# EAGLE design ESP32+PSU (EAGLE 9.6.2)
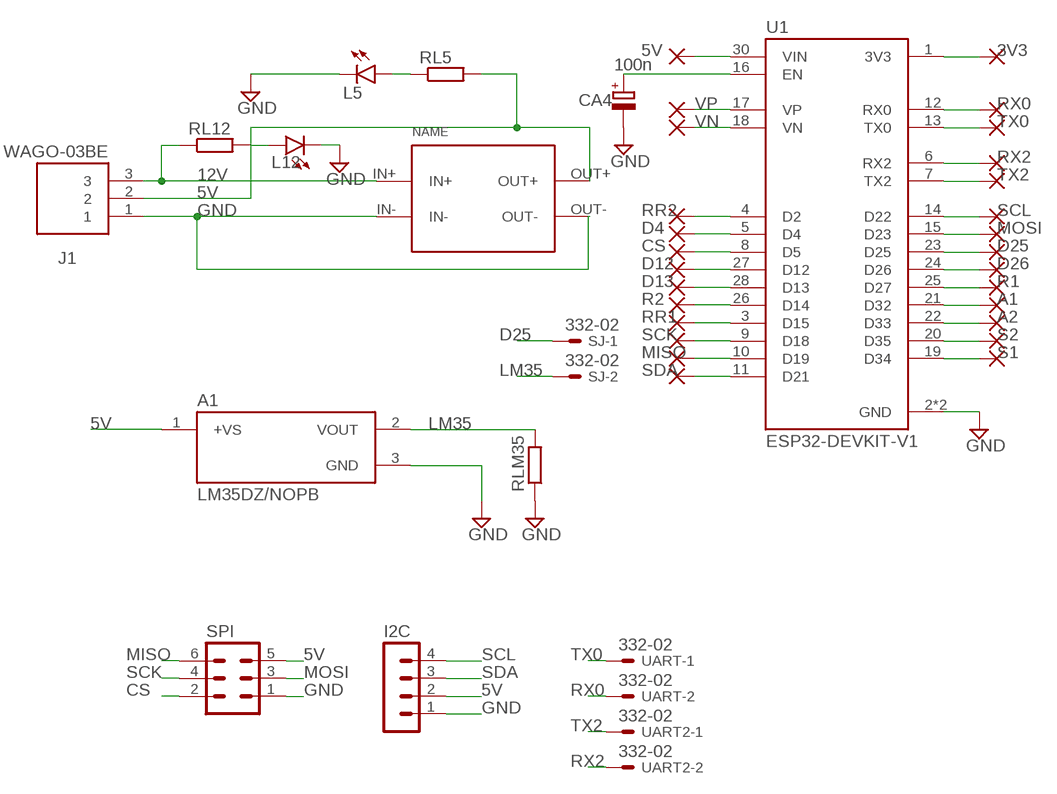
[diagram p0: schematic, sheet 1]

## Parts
A1  LM35DZ/NOPB  [TO92127P521H735-3]
CA4  100n  CPOL-EUE5-6  [E5-6]
I2C  MA04-1  [MA04-1]
J1  WAGO-03BE  [CUI_TB006-508-03BE]
L5  LED3MM  [LED3MM]
L12  LED3MM  [LED3MM]
PAD1  WIREPAD1,6/0,9  [1,6/0,9]
PAD2  WIREPAD1,6/0,9  [1,6/0,9]
PAD3  WIREPAD1,6/0,9  [1,6/0,9]
PAD4  WIREPAD1,6/0,9  [1,6/0,9]
PAD5  WIREPAD1,6/0,9  [1,6/0,9]
PAD6  WIREPAD1,6/0,9  [1,6/0,9]
PAD7  WIREPAD1,6/0,9  [1,6/0,9]
PAD8  WIREPAD1,6/0,9  [1,6/0,9]
PAD9  WIREPAD1,6/0,9  [1,6/0,9]
PAD10  WIREPAD1,6/0,9  [1,6/0,9]
PAD11  WIREPAD1,6/0,9  [1,6/0,9]
PAD12  WIREPAD1,6/0,9  [1,6/0,9]
PAD13  WIREPAD1,6/0,9  [1,6/0,9]
PAD14  WIREPAD1,6/0,9  [1,6/0,9]
PAD15  WIREPAD1,6/0,9  [1,6/0,9]
PAD16  WIREPAD1,6/0,9  [1,6/0,9]
PAD17  WIREPAD1,6/0,9  [1,6/0,9]
PAD18  WIREPAD1,6/0,9  [1,6/0,9]
PAD19  WIREPAD1,6/0,9  [1,6/0,9]
PAD20  WIREPAD1,6/0,9  [1,6/0,9]
PAD21  WIREPAD1,6/0,9  [1,6/0,9]
PAD22  WIREPAD1,6/0,9  [1,6/0,9]
PAD23  WIREPAD1,6/0,9  [1,6/0,9]
PAD24  WIREPAD1,6/0,9  [1,6/0,9]
PAD25  WIREPAD1,6/0,9  [1,6/0,9]
PAD26  WIREPAD1,6/0,9  [1,6/0,9]
PAD52  WIREPAD1,6/0,9  [1,6/0,9]
RL5  R-EU_0309/12  [0309/12]
RL12  R-EU_0309/12  [0309/12]
RLM35  R-EU_0309/12  [0309/12]
SJ  332-02  [332-02]
SPI  MA03-2  [MA03-2]
U1  ESP32-DEVKIT-V1  [MODULE_ESP32_DEVKIT_V1]
U$1  CP8-ADJ  [CP8-ADJ]
UART  332-02  [332-02]
UART2  332-02  [332-02]

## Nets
3V3: PAD11.1(P) U1.1(3V3)
5V: A1.1(+VS) I2C.2 J1.2 PAD25.1(P) RL5.2 SPI.5 U1.30(VIN) U$1.OUT+
12V: J1.3 RL12.1 U$1.IN+
A1: PAD21.1(P) U1.21(D32)
A2: PAD22.1(P) U1.22(D33)
CS: PAD3.1(P) SPI.2 U1.8(D5)
D4: PAD2.1(P) U1.5(D4)
D12: PAD4.1(P) U1.27(D12)
D13: PAD5.1(P) U1.28(D13)
D25: PAD18.1(P) SJ.1 U1.23(D25)
D26: PAD19.1(P) U1.24(D26)
GND: A1.3(GND) CA4.- I2C.1 J1.1 L5.K(C) L12.K(C) RLM35.1 SPI.1 U1.2(GND) U1.29(GND) U$1.IN- U$1.OUT-
LM35: A1.2(VOUT) RLM35.2 SJ.2
MISO: PAD9.1(P) SPI.6 U1.10(D19)
MOSI: PAD17.1(P) SPI.3 U1.15(D23)
N$14: L12.A RL12.2
N$23: L5.A RL5.1
N$25: CA4.+ U1.16(EN)
R1: PAD20.1(P) U1.25(D27)
R2: PAD6.1(P) U1.26(D14)
RR1: PAD7.1(P) U1.3(D15)
RR2: PAD1.1(P) U1.4(D2)
RX0: PAD12.1(P) U1.12(RX0) UART.2
RX2: PAD14.1(P) U1.6(RX2) UART2.2
S1: PAD24.1(P) U1.19(D34)
S2: PAD23.1(P) U1.20(D35)
SCK: PAD8.1(P) SPI.4 U1.9(D18)
SCL: I2C.4 PAD16.1(P) U1.14(D22)
SDA: I2C.3 PAD10.1(P) U1.11(D21)
TX0: PAD13.1(P) U1.13(TX0) UART.1
TX2: PAD15.1(P) U1.7(TX2) UART2.1
VN: PAD52.1(P) U1.18(VN)
VP: PAD26.1(P) U1.17(VP)

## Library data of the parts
A1 = LM35DZ_NOPB:LM35DZ/NOPB; CHECK_PRICES: https://www.snapeda.com/parts/LM35DZ/NOPB/Texas+Instruments/view-part/?ref=eda; DESCRIPTION: 1C high voltage analog temperature sensor, 10 mV/C; DIGIKEY_PART_NUMBER: LM35DZ/NOPB-ND; MF: Texas; MP: LM35DZ/NOPB; PACKAGE: None; SNAPEDA_LINK: https://www.snapeda.com/parts/LM35DZ/NOPB/Texas+Instruments/view-part/?ref=snap
CA4 = rcl-ws:CPOL-EU: POLARIZED CAPACITOR, European symbol; SPICEPREFIX: C
I2C = con-lstb:MA04-1: PIN HEADER; OC_FARNELL: unknown; OC_NEWARK: unknown
J1 = TB006-508-03BE:WAGO-03BE: Check availability; AVAILABILITY: In Stock; CHECK_PRICES: https://www.snapeda.com/parts/TB006-508-03BE/Same+Sky/view-part/?ref=eda; DESCRIPTION: 2~24 Poles, Screw Type, Horizontal, 5.08 Pitch, 26~14 (AWG), Terminal Block Connector; MF: Same Sky; MP: TB006-508-03BE; PACKAGE: None; PRICE: None; SNAPEDA_LINK: https://www.snapeda.com/parts/TB006-508-03BE/Same+Sky/view-part/?ref=snap
L5 L12 = led_WS:LED: LED
PAD1-PAD26 PAD52 = wirepad-ws:WIREPAD: Wire PAD connect wire on PCB
RL5 RL12 RLM35 = rcl-ws:R-EU_: RESISTOR, European symbol; SPICEPREFIX: R
SJ UART UART2 = con-garry-ws:332-02: 2 Pin - 2mm Dual Row
SPI = con-lstb-ws:MA03-2: PIN HEADER; OC_FARNELL: unknown; OC_NEWARK: unknown
U1 = ESP32-DEVKIT-V1:ESP32-DEVKIT-V1: Dual core, Wi-Fi: 2.4 GHz up to 150 Mbits/s,BLE (Bluetooth Low Energy) and legacy Bluetooth, 32 bits, Up to 240 MHz Check availability; AVAILABILITY: Not in stock; CHECK_PRICES: https://www.snapeda.com/parts/ESP32-DEVKIT-V1/Do+it/view-part/?ref=eda; DESCRIPTION: Dual core, Wi-Fi: 2.4 GHz up to 150 Mbits/s,BLE (Bluetooth Low Energy) and legacy Bluetooth, 32 bits, Up to 240 MHz; MF: Do it; MP: ESP32-DEVKIT-V1; PACKAGE: None; PRICE: None; SNAPEDA_LINK: https://www.snapeda.com/parts/ESP32-DEVKIT-V1/Do+it/view-part/?ref=snap
U$1 = userlib:CP8-ADJ: Voltage regulator IN: 7-35V OUT: ADJ

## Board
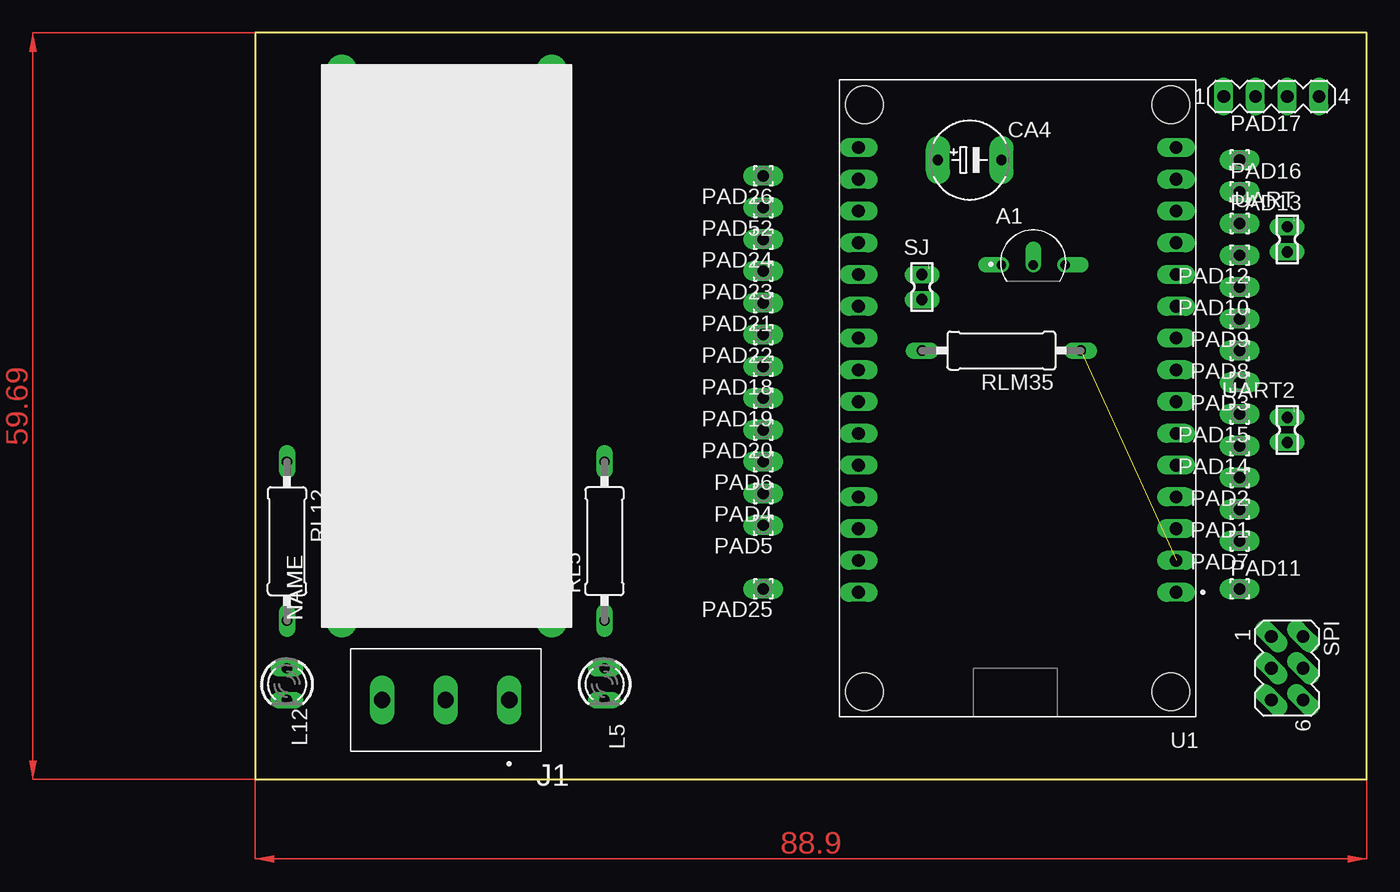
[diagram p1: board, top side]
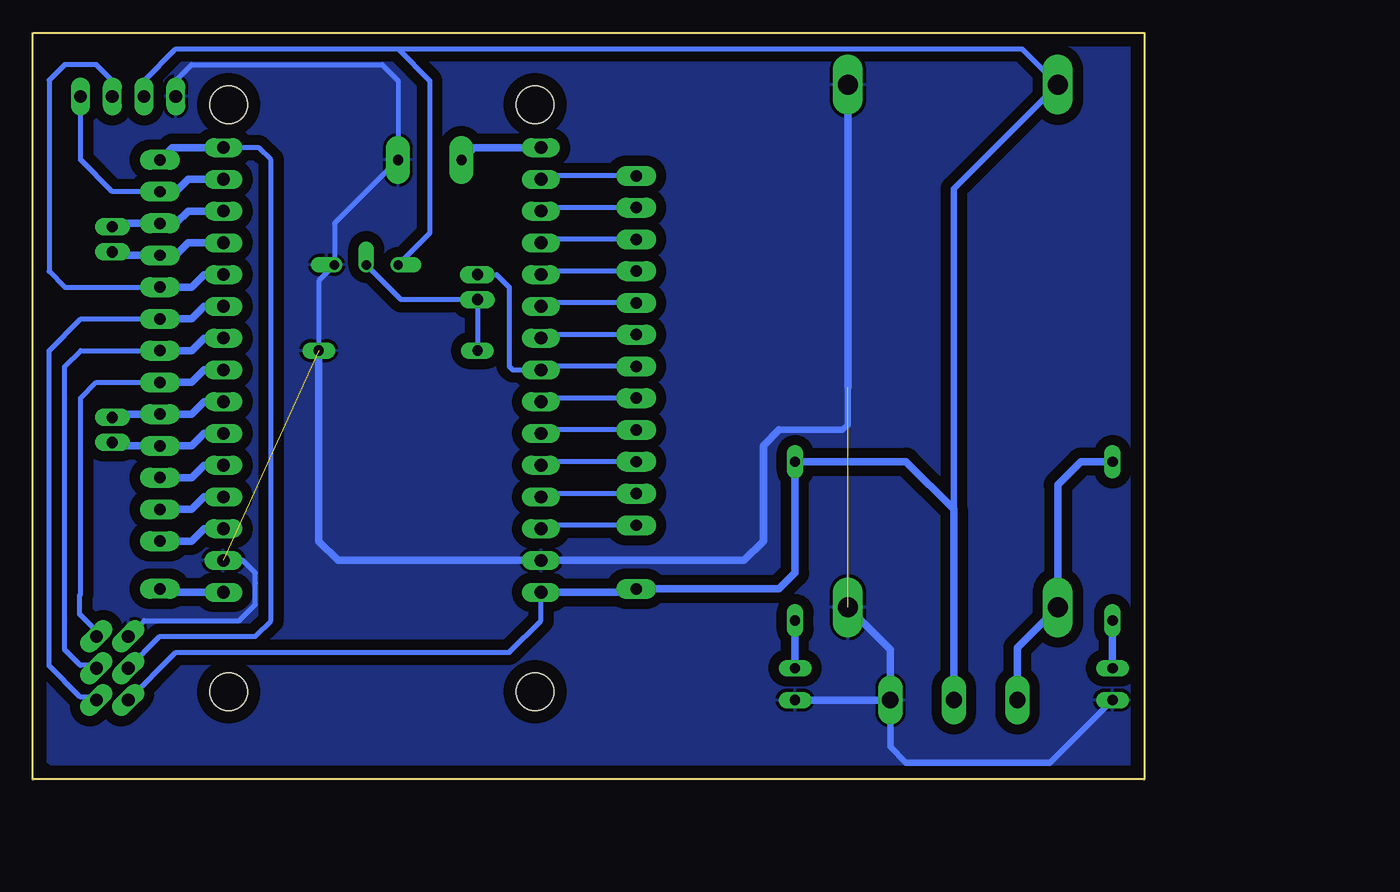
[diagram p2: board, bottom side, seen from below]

Size 88.9 x 59.69 mm. Coordinates in mm from the lower left corner, seen from the top.
Outline: 0,59.69 0,0 88.9,0 88.9,59.69 0,59.69
Copper layers (1*16): Top 0.035mm / dielectric 1.5mm / Bottom 0.035mm
Design rules "default *": minimum track width 16mil, minimum drill 0.35mm, track to track 32mil, track to pad 32mil, pad to pad 32mil, via to via 32mil, smd to smd 6mil, copper to edge 40mil, drill to drill 6mil, minimum pad ring 10mil, minimum via ring 8mil, stop-mask expansion 4mil, vias tented up to drill 0mil, thermal gap 10mil

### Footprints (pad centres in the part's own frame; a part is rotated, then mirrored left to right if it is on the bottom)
TO92127P521H735-3 = drill 0.75 pad 0.813 offset: 1 -2.54,-0.775; 2 0,-0.775; 3 2.54,-0.775
E5-6 = drill 0.813 pad 1.905 long: + -2.54,0; - 2.54,0
MA04-1 = drill 1.016 long: 1 -3.81,0; 2 -1.27,0; 3 1.27,0; 4 3.81,0
CUI_TB006-508-03BE = drill 1.3 long: 1 0,0; 2 5.08,0; 3 10.16,0
LED3MM = drill 0.813 long: A -1.27,0; K 1.27,0
1,6/0,9 = drill 0.914 pad 1.6 long: 1 0,0
0309/12 = drill 0.813 long: 1 -6.35,0; 2 6.35,0
332-02 = drill 0.9 pad 1.016 long: 1 0,-1; 2 0,1
MA03-2 = drill 1.016 pad 1.016 long: 1 -2.54,-1.27; 2 -2.54,1.27; 3 0,-1.27; 4 0,1.27; 5 2.54,-1.27; 6 2.54,1.27
MODULE_ESP32_DEVKIT_V1 = drill 1.02 pad 1.27 long: 1 -12.7,15.515; 2 -12.7,12.975; 3 -12.7,10.435; 4 -12.7,7.895; 5 -12.7,5.355; 6 -12.7,2.815; 7 -12.7,0.275; 8 -12.7,-2.265; 9 -12.7,-4.805; 10 -12.7,-7.345; 11 -12.7,-9.885; 12 -12.7,-12.425; 13 -12.7,-14.965; 14 -12.7,-17.505; 15 -12.7,-20.045; 16 12.7,-20.045; 17 12.7,-17.505; 18 12.7,-14.965; 19 12.7,-12.425; 20 12.7,-9.885; 21 12.7,-7.345; 22 12.7,-4.805; 23 12.7,-2.265; 24 12.7,0.275; 25 12.7,2.815; 26 12.7,5.355; 27 12.7,7.895; 28 12.7,10.435; 29 12.7,12.975; 30 12.7,15.515 | hole 3: -12.28,-23.475; 12.23,-23.475; 12.23,23.475; -12.28,23.475
CP8-ADJ = drill 1.6 long: IN+ -21.81,7.05; IN- -21.81,-9.75; OUT+ 19.99,7.05; OUT- 19.99,-9.75

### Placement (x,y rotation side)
A1  62.23,41.91 0 top
CA4  57.15,49.53 0 top
I2C  81.28,54.61 0 top
J1  20.32,6.35 180 top
L5  27.94,7.62 270 top
L12  2.54,7.62 270 top
PAD1  78.74,21.59 180 top
PAD2  78.74,24.13 180 top
PAD3  78.74,31.75 180 top
PAD4  40.64,22.86 180 top
PAD5  40.64,20.32 180 top
PAD6  40.64,25.4 180 top
PAD7  78.74,19.05 180 top
PAD8  78.74,34.29 180 top
PAD9  78.74,36.83 180 top
PAD10  78.74,39.37 180 top
PAD11  78.74,15.24 0 top
PAD12  78.74,41.91 180 top
PAD13  78.74,44.45 0 top
PAD14  78.74,26.67 180 top
PAD15  78.74,29.21 180 top
PAD16  78.74,46.99 0 top
PAD17  78.74,49.53 0 top
PAD18  40.64,33.02 180 top
PAD19  40.64,30.48 180 top
PAD20  40.64,27.94 180 top
PAD21  40.64,38.1 180 top
PAD22  40.64,35.56 180 top
PAD23  40.64,40.64 180 top
PAD24  40.64,43.18 180 top
PAD25  40.64,15.24 180 top
PAD26  40.64,48.26 180 top
PAD52  40.64,45.72 180 top
RL5  27.94,19.05 90 top
RL12  2.54,19.05 270 top
RLM35  59.69,34.29 180 top
SJ  53.34,39.37 180 top
SPI  82.55,8.89 270 top
U1  60.96,30.48 180 top
U$1  13.97,35.56 90 top
UART  82.55,43.18 180 top
UART2  82.55,27.94 180 top

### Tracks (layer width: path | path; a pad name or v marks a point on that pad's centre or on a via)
3V3
  Bottom 0.61: U1.1 78.47,14.96 PAD11.1
5V
  Bottom 0.406: SPI.5 77.47,10.16 50.8,10.16 48.26,12.7 U1.30 | I2C.2 80.01,55.88 77.47,58.42 59.69,58.42 | 59.69,58.42 57.15,55.88 57.15,43.67 A1.1 | 59.69,58.42 9.79,58.42 U$1.OUT+
  Bottom 0.508: U$1.OUT+ 15.24,47.23 15.24,21.59
  Bottom 0.61: U1.30 40.91,14.96 PAD25.1 29.21,15.24 27.94,16.51 RL5.2 19.05,25.4 15.24,21.59 J1.2
12V
  Bottom 0.61: J1.3 10.16,10.51 U$1.IN+ 6.92,23.56 5.08,25.4 RL12.1
A1
  Bottom 0.406: PAD21.1 48.26,38.1 U1.21
A2
  Bottom 0.406: PAD22.1 47.98,35.56 U1.22
CS
  Bottom 0.406: SPI.2 83.82,11.87 85.17,13.22 85.17,14.72 85.09,14.8 85.09,30.48 83.82,31.75 PAD3.1
  Bottom 0.61: U1.8 75.2,32.74 76.2,31.75 PAD3.1
D4
  Bottom 0.61: U1.5 75.2,25.12 76.2,24.13 PAD2.1
D12
  Bottom 0.406: PAD4.1 47.98,22.86 U1.27
D13
  Bottom 0.406: PAD5.1 47.98,20.32 U1.28
D25
  Bottom 0.406: SJ.1 51.8,40.37 50.8,39.37 50.8,38.57 50.81,38.56 50.81,34.55 50.8,34.54 50.8,33.02 50.52,32.74 U1.23 47.98,33.02 PAD18.1
D26
  Bottom 0.406: PAD19.1 47.98,30.48 U1.24
GND  (2 unrouted)
  Bottom 0.406: SPI.1 80.01,12.7 72.39,12.7 71.11,13.98 71.11,15.7 71.12,15.71 71.12,16.51 72.11,17.5 U1.2 | 65.79,34.29 RLM35.1 66.04,39.87 A1.3 64.77,44.45 CA4.- 59.69,55.88 60.96,57.15 76.2,57.15 77.47,55.88 I2C.1
  Bottom 0.508: L12.K 7.54,1.35 19.05,1.35 20.32,2.62 J1.1 | 23.72,31.75 23.72,28.35 24.13,27.94 29.21,27.94
  Bottom 0.61: U$1.IN- 20.32,10.35 J1.1 L5.K | 29.21,27.94 30.48,26.67 30.48,19.05 32.02,17.5 U1.29 64.5,17.5 66.04,19.05 RLM35.1 | U$1.OUT- 23.72,31.75 23.72,31.34
  pour Bottom: 1.27,59.69 87.63,59.69 88.9,58.42 88.9,2.54 86.36,0 1.27,0 0,1.27 0,58.42
LM35
  Bottom 0.406: RLM35.2 SJ.2 59.47,38.37 A1.2
MISO
  Bottom 0.406: SPI.6 84.04,6.57 85.09,6.57 87.61,9.08 87.61,34.29 85.06,36.83 PAD9.1
  Bottom 0.61: U1.10 75.2,37.83 76.2,36.83 PAD9.1
MOSI
  Bottom 0.406: SPI.3 78.74,11.43 71.12,11.43 69.85,12.7 69.85,49.53 70.84,50.52 U1.15
  Bottom 0.61: U1.15 77.75,50.52 PAD17.1
N$14
  Bottom 0.61: RL12.2 L12.A
N$23
  Bottom 0.61: L5.A RL5.1
N$25
  Bottom 0.61: U1.16 53.62,50.52 CA4.+
R1
  Bottom 0.406: PAD20.1 47.98,27.94 U1.25
R2
  Bottom 0.406: PAD6.1 47.98,25.4 U1.26
RR1
  Bottom 0.61: U1.3 75.2,20.05 76.2,19.05 PAD7.1
RR2
  Bottom 0.61: U1.4 75.2,22.59 76.2,21.59 PAD1.1
RX0
  Bottom 0.61: UART.2 82.28,41.91 PAD12.1 77.47,41.91 76.47,42.91 U1.12
RX2
  Bottom 0.61: UART2.2 82.28,26.67 80.01,26.67 PAD14.1 76.2,26.67 75.2,27.66 U1.6
S1
  Bottom 0.406: PAD24.1 47.98,43.18 U1.19
S2
  Bottom 0.406: PAD23.1 47.98,40.64 U1.20
SCK
  Bottom 0.406: SPI.4 84.04,9.11 85.09,9.11 86.36,10.38 86.36,33.02 85.09,34.29 PAD8.1
  Bottom 0.61: U1.9 75.2,35.28 76.2,34.29 PAD8.1
SCL
  Bottom 0.406: PAD16.1 82.55,46.99 85.09,49.53 I2C.4
  Bottom 0.61: U1.14 76.47,47.98 77.47,46.99 PAD16.1
SDA
  Bottom 0.406: I2C.3 82.55,55.88 83.82,57.15 86.36,57.15 87.61,55.91 87.61,40.62 86.36,39.37 PAD10.1
  Bottom 0.61: U1.11 75.2,40.37 76.2,39.37 PAD10.1
TX0
  Bottom 0.61: U1.13 76.47,45.45 77.47,44.45 PAD13.1 82.28,44.45 UART.1
TX2
  Bottom 0.406: UART2.1 82.55,28.66
  Bottom 0.61: U1.7 75.2,30.2 76.2,29.21 PAD15.1 82.28,29.21 UART2.1
VN
  Bottom 0.406: PAD52.1 47.98,45.72 U1.18
VP
  Bottom 0.406: PAD26.1 47.98,48.26 U1.17
(copper drawn outside any net)
  shapes: Top area x2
